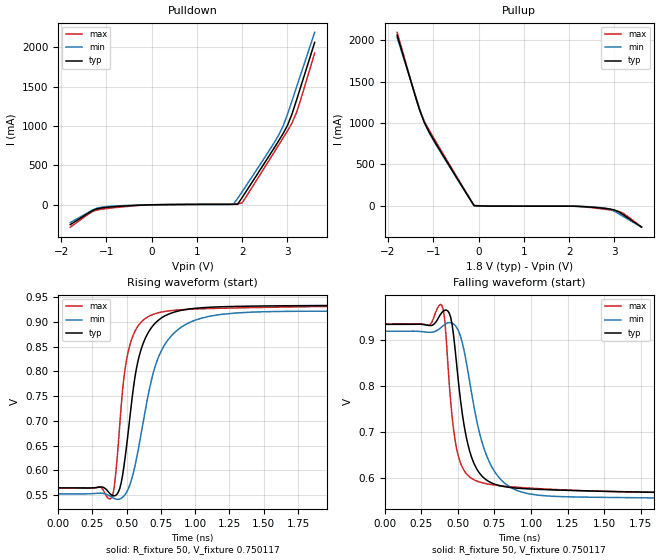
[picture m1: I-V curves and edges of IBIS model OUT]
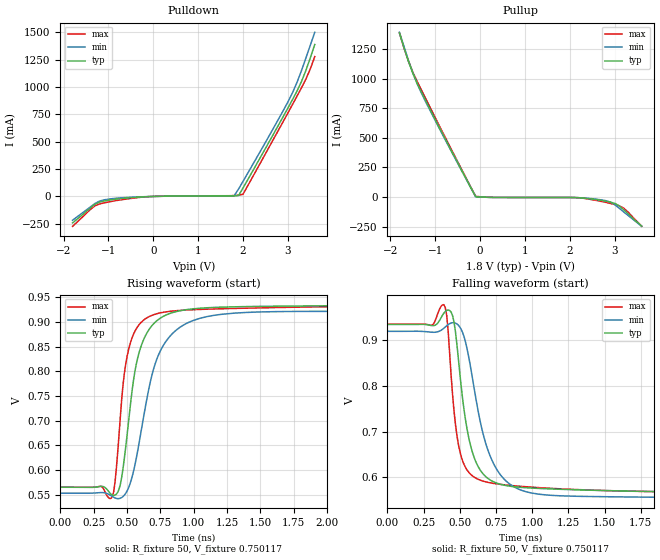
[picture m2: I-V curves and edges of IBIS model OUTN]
|   IBIS File of SG2520VGN E
|   LVDS, Vcc=1.8V, Io=3.5mA, fo<=212.5MHz
[IBIS Ver]   3.2
[File Name]   sg2520vgn_35m_18v.ibs
[File Rev]   1.0
[Date]   Sep. 11, 2020
[Source]
Fairchild Ensigna Lab's Method
[Notes]
Created by Minoru Kozaki
[Disclaimer]
Seiko Epson Corporation makes no warranty with respect to the
information contained herein.
[Copyright]
Copyright(C) 2020, Seiko Epson Corporation. All rights reserved.
|   Component
[Component]   SG2520VGN
[Manufacturer]  Seiko Epson Corporation
[Package]
R_pkg   17.7m   NA   NA
L_pkg   235p   NA   NA
C_pkg   208f   NA   NA
[Pin]   signal_name   model_name   R_pin   L_pin   C_pin
1   OE/ST   NC
2   NC   NC
3   GND   GND
4   OUT   OUT   17.7m   235p   208f
5   OUTN   OUTN   10.4m   129p   221f
6   VCC   POWER
[Diff Pin] inv_pin  vdiff  tdelay_typ
4   5   0   0
| Models and submodels in the file (2): OUT (Output), OUTN (Output)
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|   Model OUT
[Model]   OUT
Model_type   Output
Polarity   Non-Inverting
Vref = 0.75
Vmeas = 0.75
Rref = 50
Cref = 0
C_comp   4.5p   4.5p   4.5p
[Temperature Range]   25   105   -40
[Voltage Range]   1.8   1.71   1.89
[Pullup Reference]   1.8   1.71   1.89
[Pulldown Reference]   0   0   0
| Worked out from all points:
|   slope of the pulldown table from 0 to 0.27 V, typ, clamps not added: 118 ohm
|   slope of the pullup table from 0 to 0.27 V, typ, clamps not added: 78.3 ohm
|   falling waveform, R_fixture 50, V_fixture 0.750117: 20-80 % time 113ps typ, 167ps min, 81.9ps max; typ from 0.935 V to 0.565 V
|   rising waveform, R_fixture 50, V_fixture 0.750117: 20-80 % time 132ps typ, 189ps min, 97.1ps max; typ from 0.564 V to 0.934 V
[Pullup]
-1.8V     2.06A      2.034A     2.094A
-1.4V     1.329A     1.339A     1.328A
-1.3V     1.151A     1.166A     1.152A
-1.2V     1.007A     1.011A     1.021A
-1.1V     899.2mA    891.2mA    921.2mA
-1V       805mA      792.9mA    827.3mA
-100mV    2.741mA    1.692mA    6.495mA
2.1V      -4.391mA   -4.533mA   -4.229mA
2.8V      -31.03mA   -28.12mA   -40.93mA
3V        -49.05mA   -63.49mA   -57.07mA
3.2V      -108.4mA   -128.5mA   -89.88mA
3.6V      -256mA     -256.8mA   -253.7mA
[Pulldown]
-1.8V     -252.2mA   -225.8mA   -284.2mA
-1.3V     -70.15mA   -64.6mA    -83.14mA
-1.1V     -39.47mA   -29.87mA   -56.03mA
-100mV    -1.574mA   -1.248mA   -1.862mA
1.8V      6.081mA    5.271mA    8.017mA
1.9V      7.561mA    81.78mA    11.71mA
2V        94.31mA    167.8mA    24.66mA
2.8V      808.9mA    880.5mA    755.7mA
2.9V      902.4mA    997.2mA    847.4mA
3V        1.009A     1.15A      940.4mA
3.2V      1.332A     1.496A     1.174A
3.6V      2.064A     2.193A     1.929A
[Falling Waveform]
R_fixture = 50
V_fixture = 0.750117
V_fixture_min = 0.736304
V_fixture_max = 0.750507
0s        934.7mV    919.7mV    935.4mV
390ps     960.6mV    929.5mV    976.5mV
410ps     965.6mV    934.6mV    942.9mV
450ps     950.2mV    938.4mV    766.9mV
490ps     850.5mV    928.6mV    664.7mV
560ps     684.2mV    847mV      608mV
660ps     605.3mV    683mV      589.6mV
800ps     581.7mV    593.9mV    582.3mV
1.05ns    574.8mV    562.1mV    576.4mV
4ns       564.8mV    553mV      564.6mV
[Rising Waveform]
R_fixture = 50
V_fixture = 0.750117
V_fixture_min = 0.736304
V_fixture_max = 0.750507
0s        564.5mV    552.5mV    564.4mV
380ps     552.4mV    547.7mV    542.2mV
440ps     556.1mV    541.4mV    655.1mV
480ps     607mV      547.9mV    786.3mV
520ps     697.4mV    568mV      849.2mV
590ps     828.8mV    649.7mV    893.9mV
700ps     894.7mV    802.4mV    915.5mV
880ps     921.9mV    885.4mV    923.9mV
1.2ns     930.4mV    915.2mV    927.4mV
4ns       934.4mV    920mV      934.9mV
[Ramp]
R_load = 50
dV/dt_r   0.22226/132.64p   0.21974/188.14p   0.22318/98.24p
dV/dt_f   0.22226/113.37p   0.21974/166.84p   0.22318/81.87p
|   Model OUTN
[Model]   OUTN
Model_type   Output
Polarity   Inverting
Vref = 0.75
Vmeas = 0.75
Rref = 50
Cref = 0
C_comp   4.5p   4.5p   4.5p
[Temperature Range]   25   105   -40
[Voltage Range]   1.8   1.71   1.89
[Pullup Reference]   1.8   1.71   1.89
[Pulldown Reference]   0   0   0
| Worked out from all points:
|   slope of the pulldown table from 0 to 0.27 V, typ, clamps not added: 118 ohm
|   slope of the pullup table from 0 to 0.27 V, typ, clamps not added: 78.4 ohm
|   falling waveform, R_fixture 50, V_fixture 0.750117: 20-80 % time 115ps typ, 167ps min, 84.1ps max; typ from 0.935 V to 0.566 V
|   rising waveform, R_fixture 50, V_fixture 0.750117: 20-80 % time 132ps typ, 189ps min, 98.2ps max; typ from 0.565 V to 0.934 V
[Pullup]
-1.8V     1.387A     1.393A     1.388A
-1.6V     1.148A     1.157A     1.15A
-1.5V     1.045A     1.049A     1.055A
-1.3V     879.3mA    870.8mA    897.3mA
-800mV    507mA      499.7mA    520.2mA
-100mV    2.73mA     1.686mA    6.492mA
2.1V      -4.39mA    -4.568mA   -4.227mA
2.7V      -28.16mA   -24.32mA   -37.34mA
2.9V      -42.9mA    -42.57mA   -53.94mA
3V        -53.71mA   -64.32mA   -63.59mA
3.2V      -108.2mA   -125.8mA   -93.56mA
3.6V      -246.2mA   -247.7mA   -246.6mA
[Pulldown]
-1.8V     -242.2mA   -217.5mA   -273.1mA
-1.3V     -71.45mA   -64.54mA   -85.61mA
-900mV    -28.51mA   -19.78mA   -42.75mA
-100mV    -1.551mA   -1.234mA   -1.826mA
1.8V      6.059mA    5.256mA    7.979mA
1.9V      7.525mA    67.07mA    11.63mA
2V        77.07mA    137.5mA    19.84mA
2.8V      659.1mA    713.2mA    613.1mA
3.1V      882.6mA    945.1mA    838.2mA
3.3V      1.047A     1.146A     989.9mA
3.5V      1.266A     1.382A     1.165A
3.6V      1.389A     1.501A     1.278A
[Falling Waveform]
R_fixture = 50
V_fixture = 0.750117
V_fixture_min = 0.736304
V_fixture_max = 0.750507
0s        934.6mV    919.6mV    935.3mV
390ps     959.2mV    926.3mV    977.9mV
410ps     965.3mV    931.8mV    954.6mV
450ps     954.6mV    938.5mV    783.3mV
500ps     830.2mV    929.3mV    658.4mV
570ps     676.1mV    850.2mV    608.7mV
660ps     608.4mV    697.1mV    592.2mV
800ps     583.6mV    598.6mV    584.2mV
1.05ns    576mV      563.4mV    577.8mV
4ns       565.6mV    553.6mV    565.5mV
[Rising Waveform]
R_fixture = 50
V_fixture = 0.750117
V_fixture_min = 0.736304
V_fixture_max = 0.750507
0s        565.2mV    553.1mV    565.2mV
380ps     551mV      548.2mV    542.7mV
430ps     555.1mV    542.1mV    636.3mV
470ps     603.8mV    546.5mV    772.9mV
520ps     719.2mV    570.3mV    852.8mV
590ps     837.4mV    654.3mV    894mV
700ps     896.2mV    805.3mV    914.3mV
880ps     921.4mV    885.5mV    922.7mV
1.2ns     929.5mV    914.9mV    926.3mV
4ns       934.3mV    919.9mV    934.7mV
[Ramp]
R_load = 50
dV/dt_r   0.22120/132.46p   0.21870/187.05p   0.22211/98.94p
dV/dt_f   0.22120/114.38p   0.21870/166.62p   0.22211/83.97p
